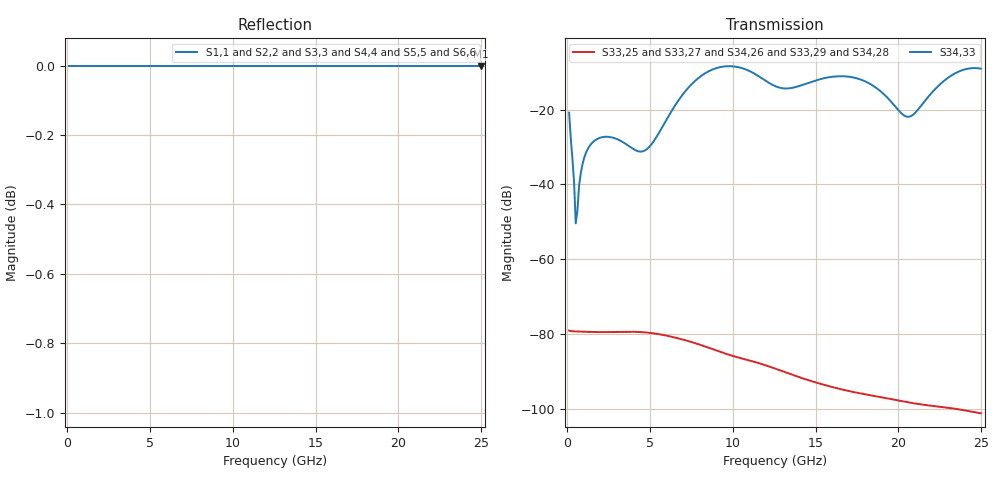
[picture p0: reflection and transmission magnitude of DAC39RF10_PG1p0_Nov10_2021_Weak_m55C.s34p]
! Touchstone Ver. 1.0
! Number of ports is 34
# Hz	S	RI	R	50.000000
! SCATTERING PARAMETERS  :
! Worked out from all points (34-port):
!   250 points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, 100 MHz to 25 GHz, reference 50 ohm
!   strongest paths, dB at 100 MHz, 6.3 GHz, 12.6 GHz, 18.8 GHz, 25 GHz:
!     S34,33: -20.8, -20.3, -13.7, -14.6, -9.0
!     S33,25: -79.1, -80.8, -89.3, -96.8, -101.2
!     S33,27: -79.1, -80.8, -89.4, -96.9, -101.4
!     S34,26: -79.1, -80.7, -89.4, -96.9, -101.5
!     S33,29: -79.1, -80.8, -89.4, -97.0, -101.6
!     S34,28: -79.1, -80.8, -89.5, -97.0, -101.7
!   lowest |S11| = 0.0 dB at 25 GHz (marker M1)
!   |S11| at or under -10 dB: nowhere
